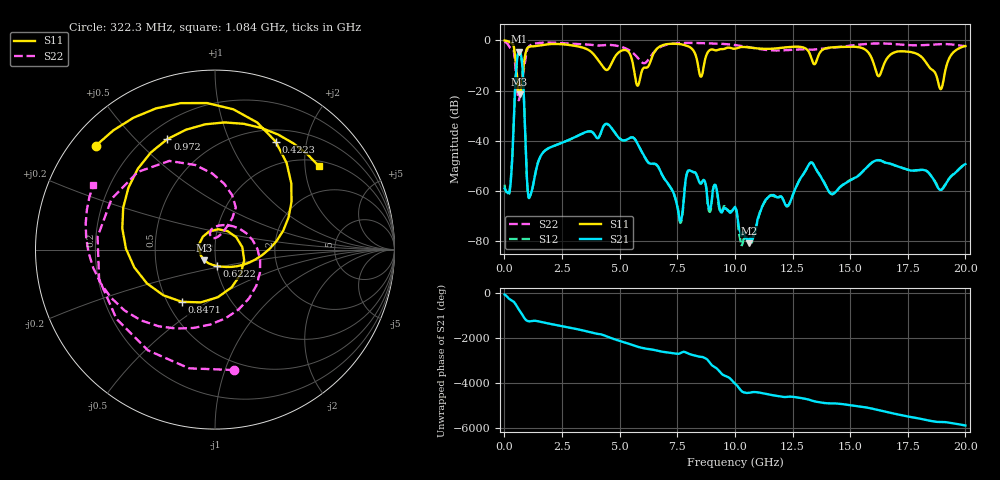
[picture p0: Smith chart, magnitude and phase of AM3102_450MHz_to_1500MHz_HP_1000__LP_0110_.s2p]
!Agilent Technologies,E8364B,MY43040894,A.07.50.67
!Agilent E8364B: A.07.50.67
!Date: Thursday, January 11, 2018 05:57:46
!Correction: S11(Full 2 Port(1,2))
!S21(Full 2 Port(1,2))
!S12(Full 2 Port(1,2))
!S22(Full 2 Port(1,2))
!S2P File: Measurements: S11, S21, S12, S22:
# Hz S  dB  R 50
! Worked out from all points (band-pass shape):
!   1601 points, 10 MHz to 20 GHz, reference 50 ohm
!   highest |S21| = -4.59 dB at 634.7 MHz (marker M1); lowest = -80.8 dB at 10.62 GHz (marker M2)
!   |S21| within 3 dB of the highest: 552 MHz to 752 MHz (200 MHz wide, 30.7 % of centre)
!   lowest |S11| = -21.5 dB at 659.7 MHz (marker M3), VSWR 1.18, Z = 44.1 - j5.26 ohm
!   |S11| at or under -10 dB: 5.589 GHz to 6.267 GHz (678 MHz wide, 11.4 % of centre); 16.05 GHz to 16.45 GHz (400.5 MHz wide, 2.47 % of centre); 18.37 GHz to 19.18 GHz (811 MHz wide, 4.32 % of centre)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
!   |S22| runs from -23.9 to -0.5 dB; largest |S21 - S12| = 0.0014
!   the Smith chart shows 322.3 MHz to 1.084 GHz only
!   S11 on the Smith chart (normalised r, x): 322.3 MHz: 0.07, +0.37; 422.3 MHz: 0.65, +1.50; 622.2 MHz: 1.01, -0.19; 847.1 MHz: 0.59, -0.39; 972 MHz: 0.28, +0.62; 1.084 GHz: 1.13, +2.36
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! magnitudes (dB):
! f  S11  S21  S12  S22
! 10 MHz  -0.1  -59.0  -57.5  -0.5
! 322.3 MHz  -1.1  -50.1  -49.6  -3.4
! 422.3 MHz  -3.2  -28.7  -28.8  -5.1
! 622.2 MHz  -20.7  -4.6  -4.6  -23.9
! 634.7 MHz  -21.3  -4.6  -4.6  -23.8
! 659.7 MHz  -21.5  -4.7  -4.7  -22.8
! 847.1 MHz  -9.2  -22.9  -22.8  -11.0
! 972 MHz  -3.5  -53.8  -54.0  -4.3
! 1.084 GHz  -2.6  -62.6  -62.7  -2.3
! 3.346 GHz  -2.8  -37.3  -37.3  -1.6
! 5.782 GHz  -18.1  -41.3  -41.3  -6.9
! 6.682 GHz  -2.9  -50.5  -50.6  -3.2
! 7.631 GHz  -1.5  -72.1  -72.8  -1.1
! 8.043 GHz  -2.7  -51.8  -51.8  -1.0
! 8.531 GHz  -14.5  -57.0  -57.0  -1.1
! 10.01 GHz  -3.4  -66.3  -66.9  -1.9
! 10.62 GHz  -2.8  -80.8  -80.3  -2.8
! 13.34 GHz  -7.8  -48.7  -48.7  -3.8
! 14.23 GHz  -2.8  -61.2  -61.4  -3.0
! 16.68 GHz  -6.3  -49.0  -49.1  -1.3
! 18.93 GHz  -19.4  -59.6  -59.5  -1.5
! 20 GHz  -2.3  -49.3  -49.3  -2.3
